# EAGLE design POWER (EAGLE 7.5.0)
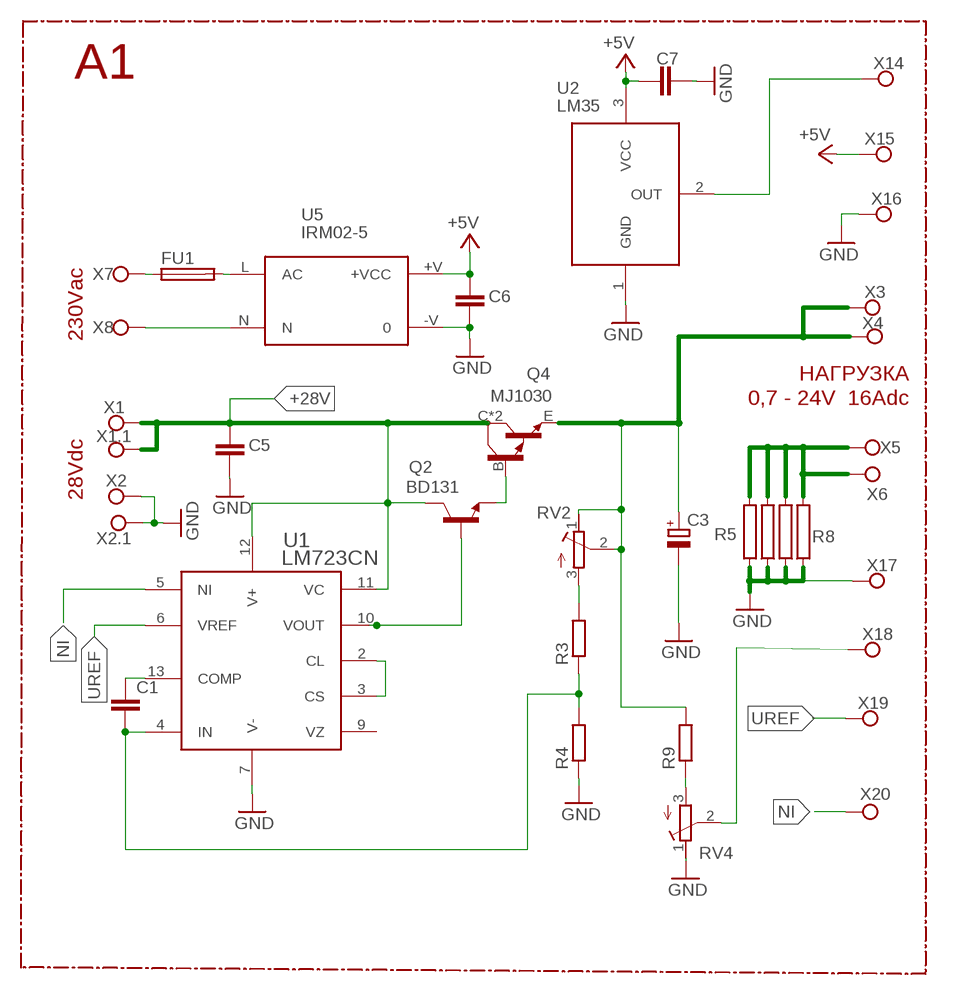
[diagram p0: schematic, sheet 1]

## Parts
C1  C-EUC1206  [C1206]
C3  CPOL-EUE35-16AXIAL  [E35-16]
C5  C-EUC1206  [C1206]
C6  C-EUC1206  [C1206]
C7  C-EUC1206  [C1206]
FU1  FUSEGSH15 1A 5x20mm  FUSEGSH15  [GSH15]
Q2  BD131  BD139  [TO126]
Q4  MJ1030  MJ3001  [TO3]
R3  R-EU_R1206  [R1206]
R4  R-EU_R1206  [R1206]
R5  RKH208-8  [KH208-8]
R6  RKH208-8  [KH208-8]
R7  RKH208-8  [KH208-8]
R8  RKH208-8  [KH208-8]
R9  R-EU_R1206  [R1206]
RV2  R-TRIMM-3386-F  [R-TRIMM-3386F]
RV4  R-TRIMM-3386-F  [R-TRIMM-3386F]
U1  LM723CN  [DIP14]
U2  LM35  [TO92]
U5  IRM02-5  IRM02  [IRM02]
X1  TPPAD1-20  [P1-20]
X1.1  TPPAD1-20  [P1-20]
X2  TPPAD1-20  [P1-20]
X2.1  TPPAD1-20  [P1-20]
X3  TPPAD1-20  [P1-20]
X4  TPPAD1-20  [P1-20]
X5  TPPAD1-20  [P1-20]
X6  TPPAD1-20  [P1-20]
X7  TPPAD1-20  [P1-20]
X8  TPPAD1-20  [P1-20]
X14  TPPAD1-20  [P1-20]
X15  TPPAD1-20  [P1-20]
X16  TPPAD1-20  [P1-20]
X17  TPPAD1-20  [P1-20]
X18  TPPAD1-20  [P1-20]
X19  TPPAD1-20  [P1-20]
X20  TPPAD1-20  [P1-20]

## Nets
+5V: C6.1 C7.2 U2.3(VCC) U5.+V(+VCC) X15.TP
+28V: C5.1 Q2.2(C) Q4.C Q4.C/(C) U1.11(VC) U1.12(V+) X1.1.TP X1.TP
GND: C3.- C5.2 C6.2 C7.1 R4.1 R5.1 R6.1 R7.1 R8.1 RV4.1(A) U1.7(V-) U2.1(GND) U5.-V X2.1.TP X2.TP X16.TP X17.TP
N$1: U2.2(OUT) X14.TP
N$2: FU1.2 U5.L(AC)
N$3: FU1.1 X7.TP
N$4: R9.1 RV4.3(E)
N$5: C1.2 R3.1 R4.2 U1.4(IN)
N$6: C1.1 U1.13(COMP)
N$7: U1.2(CL) U1.3(CS)
N$9: Q2.1(E) Q4.B
N$10: Q2.3(B) U1.10(VOUT)
N$11: C3.+ Q4.E R9.2 RV2.1(A) RV2.2(S) X3.TP X4.TP
N$12: R5.2 R6.2 R7.2 R8.2 X5.TP X6.TP
N$13: R3.2 RV2.3(E)
N$34: U5.N X8.TP
N$37: RV4.2(S) X18.TP
NI: U1.5(NI) X20.TP
UREF: U1.6(VREF) X19.TP
Unconnected: U1.9(VZ)

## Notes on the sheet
- A1
- 230Vac
- НАГРУЗКА
- 0,7 - 24V  16Adc
- 28Vdc

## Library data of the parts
C1 C5-C7 = rcl:C-EU: CAPACITOR, European symbol
C3 = rcl:CPOL-EU: POLARIZED CAPACITOR, European symbol
FU1 = fuse:FUSE: Fuse; OC_FARNELL: unknown; OC_NEWARK: unknown
Q2 = transistor-npn:BD139*: NPN Transistor
Q4 = transistor-npn:MJ3001*: NPN Darlington Transistor
R3 R4 R9 = rcl:R-EU_: RESISTOR, European symbol
R5-R8 = resistor-power:R: Power Resitor; OC_FARNELL: unknown; OC_NEWARK: unknown
RV2 RV4 = rcl:R-TRIMM-3386-F
U1 = v-reg:LM723CN: 150mA out, Voltage Regulator
U2 = transistor-neu-to92:LM35: Precision Centigrade Temperature Sensor (-55C to 150C)
U5 = acdc:IRM02: 2W Single Output ACDC converter
X1 X1.1 X2 X2.1 X3-X8 X14-X20 = testpad:TP: Test pad

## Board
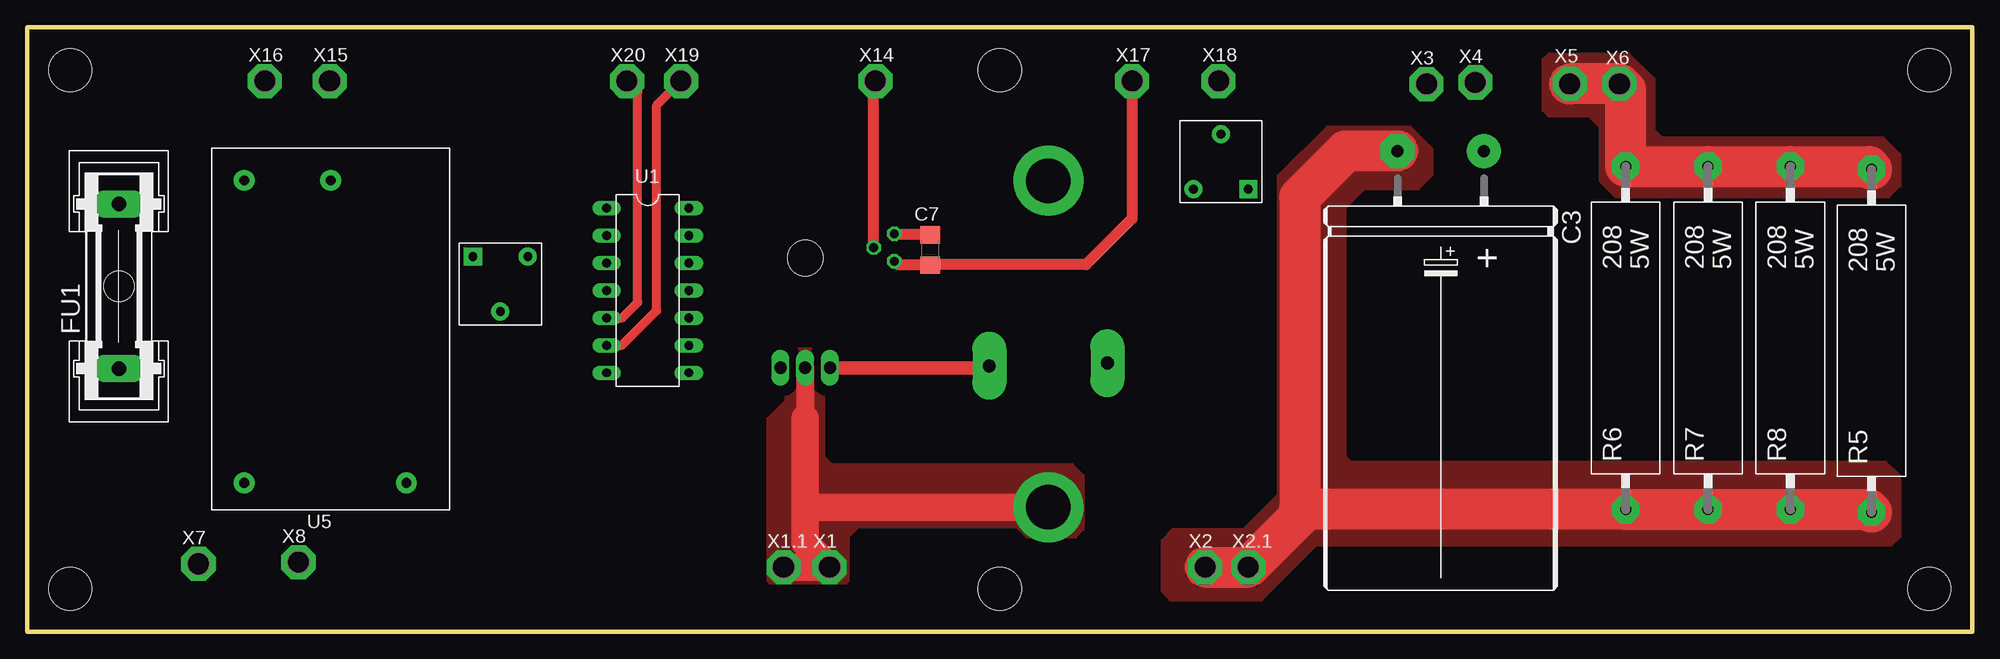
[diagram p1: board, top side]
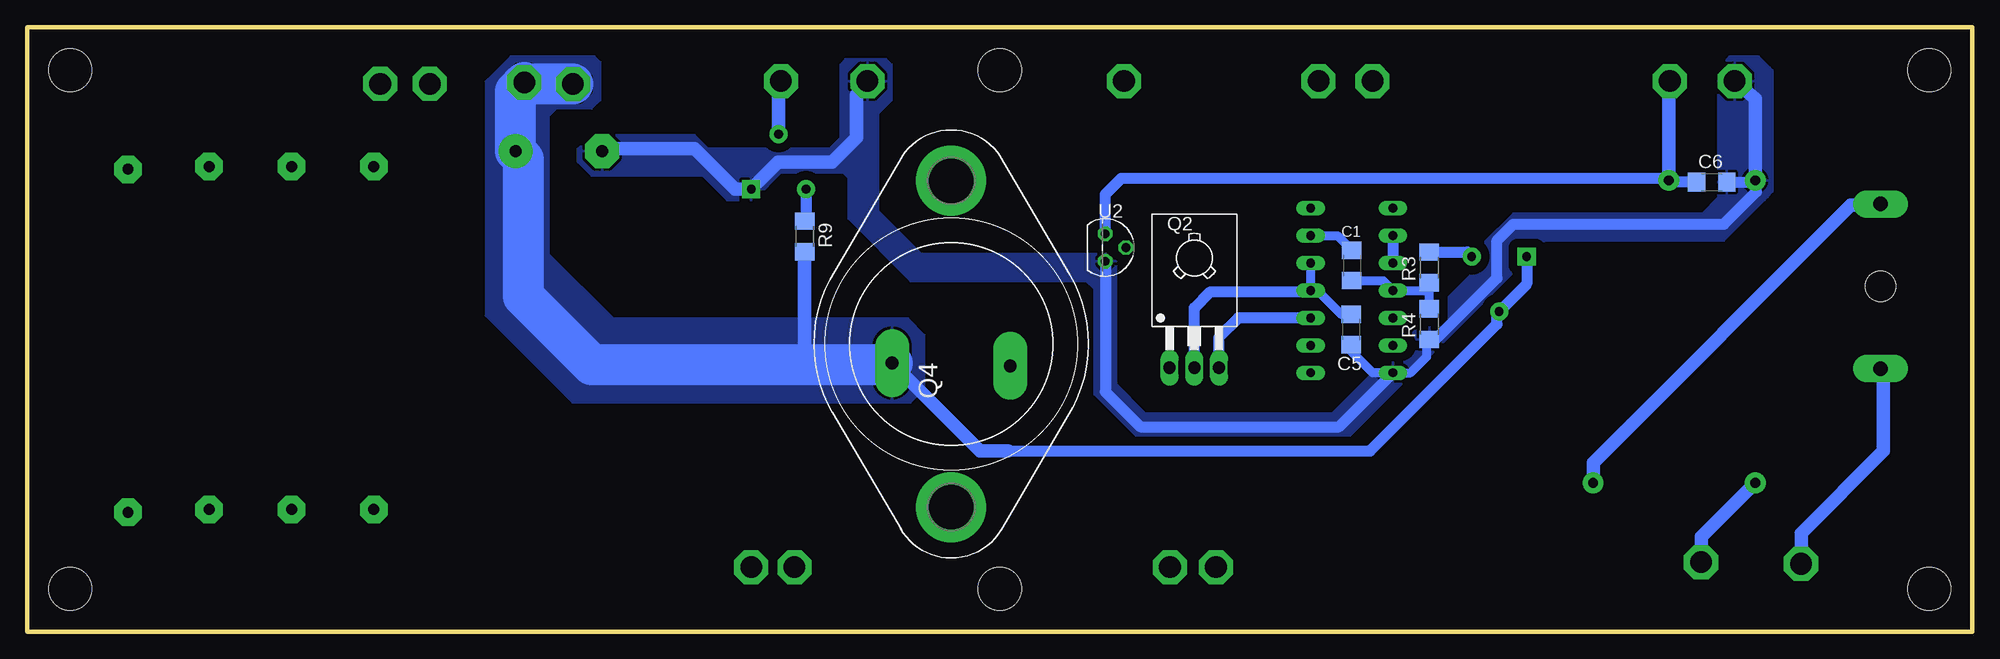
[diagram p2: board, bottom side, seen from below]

Size 180 x 56 mm. Coordinates in mm from the lower left corner, seen from the top.
Outline: 0,0 160,0
Outline: 0,0 0,56 180,56 180,0 0,0
Copper layers (1*16): Top 0.035mm / dielectric 1.5mm / Bottom 0.035mm
Design rules "default": minimum track width 10mil, minimum drill 24mil, track to track 8mil, track to pad 8mil, pad to pad 8mil, via to via 8mil, smd to smd 8mil, copper to edge 40mil, drill to drill 8mil, minimum pad ring 10mil, minimum via ring 8mil, stop-mask expansion 4mil, vias tented up to drill 0mil, thermal gap 10mil
Holes 4 mm at 4,52 4,4 90,52 90,4 176,52 176,4

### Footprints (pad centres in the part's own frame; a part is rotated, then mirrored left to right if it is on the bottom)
C1206 = smd 1.6 x 1.8: 1 -1.4,0; 2 1.4,0
E35-16 = drill 1.118 pad 3.15: + -22.86,4 | drill 1.118 pad 3.15 octagon: - -22.86,-4
GSH15 = drill 1.321 pad 2.54 long: 1 -7.62,0; 2 7.62,0 | hole 2.794: 0,0
TO126 = drill 1.118 long: 1 -2.286,-5.08; 2 0,-5.08; 3 2.286,-5.08 | hole 3.302: 0,5.08
TO3 = drill 1.194 pad 3.15 long: B -2.032,-5.461; E -1.778,5.461 | drill 4.115 pad 6.477: C 15.113,0; C/ -15.113,0
R1206 = smd 1.6 x 1.803: 1 -1.422,0; 2 1.422,0
KH208-8 = drill 1.016 pad 2.54 octagon: 1 -15.875,0; 2 15.875,0
R-TRIMM-3386F = drill 0.8 pad 1.676 square: 1 0,0 | drill 0.8 pad 1.676: 2 5.08,2.54; 3 0,5.08
DIP14 = drill 0.813 long: 1 -3.81,-3.81; 2 -1.27,-3.81; 3 1.27,-3.81; 4 3.81,-3.81; 5 6.35,-3.81; 6 8.89,-3.81; 7 11.43,-3.81; 8 11.43,3.81; 9 8.89,3.81; 10 6.35,3.81; 11 3.81,3.81; 12 1.27,3.81; 13 -1.27,3.81; 14 -3.81,3.81
TO92 = drill 0.813 octagon: 1 1.27,0; 2 0,1.905; 3 -1.27,0
IRM02 = drill 0.9 pad 1.93: +V 30.5,-11; -V 30.5,-3; L 2.5,-18; N 2.5,-3
P1-20 = drill 2.007 pad 3.15 octagon: TP 0,0

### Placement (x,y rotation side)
C1  57.42,33.93 270 bottom
C3  130.81,21.65 270 top
C5  57.5,28 270 bottom
C6  24.12,41.64 0 bottom
C7  83.59,35.37 90 top
FU1  8.5,32 90 top
Q2  72,29.54 0 bottom
Q4  94.49,26.66 90 bottom
R3  50.25,33.75 90 bottom
R4  50.25,28.5 90 bottom
R5  170.66,26.96 90 top
R6  147.91,27.21 90 top
R7  155.53,27.21 90 top
R8  163.15,27.21 90 top
R9  108.04,36.62 270 bottom
RV2  41.25,34.75 270 top
RV4  113,41 90 top
U1  57.43,35.42 270 top
U2  80.24,35.59 270 bottom
U5  17.1,11.3 90 top
X1  74.25,6 0 top
X1.1  70,6 0 top
X2  109,6 0 top
X2.1  113,6 0 top
X3  129.49,50.72 0 top
X4  133.99,50.87 0 top
X5  142.73,50.74 90 top
X6  147.33,50.74 90 top
X7  15.86,6.31 0 top
X8  25.11,6.46 0 top
X14  78.5,51 0 top
X15  28,51 0 top
X16  22,51 0 top
X17  102.25,51 0 top
X18  110.25,51 0 top
X19  60.5,51 0 top
X20  55.5,51 0 top

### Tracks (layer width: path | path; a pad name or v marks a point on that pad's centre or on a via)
+5V
  Top 1.016: C7.2 80.33,36.77 U2.3
  Bottom 1.016: U2.3 80.24,40.51 78.75,42 28.3,42 U5.+V 27.94,41.64 C6.1
  Bottom 1.27: U5.+V 28.1,50.4 X15.TP
+28V
  Top 1.676: Q2.2 72,19.75
  Top 2.54: 72,19.75 72,11.75 | 72,11.75 72,8.25 X1.TP X1.1.TP | Q4.C/ 72.2,11.55 72,11.75
  Bottom 0.813: C5.1 58.4,29.4 60.75,31.75 61.1,31.75 U1.11 U1.12
  Bottom 1.016: Q2.2 72,30 70.5,31.5 61.35,31.5 U1.11
  pour Top (isolate 1.016, no thermals): 95.5,15.5 74.5,15.5 73.75,16.25 73.75,26 73.5,26.25 71,26.25 70.75,26 70.75,23 70.25,22.5 70.25,21.5 68.5,19.75 68.5,4.75 68.75,4.5 75.75,4.5 76,4.75 76,8.75 77,9.75 91.5,9.75 92.5,8.75 97,8.75 97.75,9.5 97.75,14.5 96.75,15.5
GND
  Top 1.016: U2.1 80.59,33.97 C7.1 83.62,34 98,34 102.25,38.25 X17.TP
  Top 3.81: R5.1 170.41,11.34 R8.1 R7.1 R6.1 118.33,11.34 118.12,11.12 | 118.12,11.12 X2.1.TP X2.TP | C3.- 122.01,44.51 117.75,40.25 117.75,11.5 118.12,11.12
  Bottom 0.813: C5.2 57.5,26 55.5,24 U1.7 52.01,23.99 50.5,25.5 50.5,26.83 R4.1
  Bottom 1.016: U2.1 80.24,22.24 77,19 58.61,19 U1.7 | R4.1 49.67,27.08 44,32.75 44,36.25 42.5,37.75 23,37.75 20,40.75 20,41.7 U5.-V 20.26,41.64 C6.2
  Bottom 1.27: U5.-V 20.1,49.35 X16.TP | C3.- 126.57,44.75 118.25,44.75 114.5,41 RV4.1 110.5,43.5 105.5,43.5 103.25,45.75 103.25,49.75 X17.TP
  pour Bottom (isolate 0.813): 18.75,52.25 19.75,53.25 22.5,53.25 23.5,52.25 23.5,40.25 25,38.75 42.5,38.75 45.25,36 45.25,34.25 59.25,20.25 76.5,20.25 79.25,23 79.25,34.5 79.75,35 97.25,35 101.25,39 101.25,48 100,49.25 100,52.5 100.5,53 104.25,53 104.75,52.5 104.75,45.75 105.75,44.75 117,44.75 118.25,46 127.75,46 129,44.75 129,43.5 127.75,42.25 117.5,42.25 115.25,40 112.75,40 110.25,42.5 104.5,42.5 104,42 104,38.25 98.25,32.5 82,32.5 81.25,31.75 81.25,22 77,17.75 58,17.75 39.5,36.25 23,36.25 19.25,40 19,40.25 18.5,40.75 18.5,52
  pour Top (isolate 1.016): 106.25,9.5 112.5,9.5 115.75,12.75 115.75,42.25 120.25,46.75 128,46.75 130,44.75 130,42.25 128.75,41 123.75,41 122,39.25 122,16.25 122.5,15.75 172,15.75 173.25,14.5 173.25,8.75 172.5,8 119.25,8 114.25,3 105.75,3 105,3.75 105,8.5 106,9.5
N$1
  Top 1.016: U2.2 78.33,50.59 X14.TP
N$2
  Bottom 1.27: U5.L 35.1,15.65 11.25,39.5 7.75,39.5 7.5,39.75 8.37,39.75 FU1.2
N$3
  Bottom 1.27: X7.TP 15.86,9.14 8.25,16.75 8.25,24.13 FU1.1
N$4
  Bottom 1.016: RV4.3 107.92,38.16 R9.1
N$5
  Bottom 0.813: C1.2 54.54,32.53 U1.4 50.36,31.61 50.25,31.5 | R4.2 50.25,31.5 | 50.25,31.5 R3.1
N$6
  Bottom 0.813: U1.13 58.78,36.69 C1.1
N$7
  Bottom 1.016: U1.2 U1.3
N$9
  Top 1.27: Q2.1 88.86,24.46 Q4.B
N$10
  Bottom 1.016: U1.10 67.93,29.07 69.75,27.25 69.75,24.5 Q2.3
N$11
  Bottom 1.016: 89.25,16.75 55.75,16.75 44,28.5 44,29.46 RV2.2 41.25,32.21 RV2.1
  Bottom 1.27: R9.2 108.04,24.79 108,24.75 | 89.25,16.75 91.82,16.75 Q4.E
  Bottom 3.81: Q4.E 100.08,24.75 108,24.75 127.75,24.75 134.06,31.06 134.06,43.76 C3.+ 134.81,50.05 X4.TP 133.84,50.72 X3.TP
  pour Bottom (isolate 1.016): 127.5,53.25 135.25,53.25 137.5,51 137.5,29.25 129.5,21.25 98.25,21.25 97,22.5 97,27.5 98.5,29 125.75,29 131.75,35 131.75,47.75 131,48.5 127.75,48.5 127,49.25 127,52.75
N$12
  Top 3.81: X5.TP X6.TP 147.91,50.16 R6.2 R7.2 R8.2 170.41,43.09 R5.2
  pour Top (isolate 1.016): 140.25,53 140.75,53.5 148.25,53.5 150.5,51.25 150.5,46.5 151.25,45.75 171.75,45.75 173.25,44.25 173.25,41.25 172.25,40.25 147,40.25 145.5,41.75 145.5,46.75 144.5,47.75 140.75,47.75 140.25,48.25 140.25,52.75
N$13
  Bottom 1.016: R3.2 46.75,35.17 RV2.3
N$34
  Bottom 1.27: X8.TP 25.11,8.79 U5.N
N$37
  Bottom 1.27: RV4.2 110.46,50.29 X18.TP
NI
  Top 0.813: U1.5 55.07,29.07 56.5,30.5 56.5,50 X20.TP
UREF
  Top 0.813: U1.6 55.03,26.53 58.25,29.75 58.25,48.75 X19.TP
